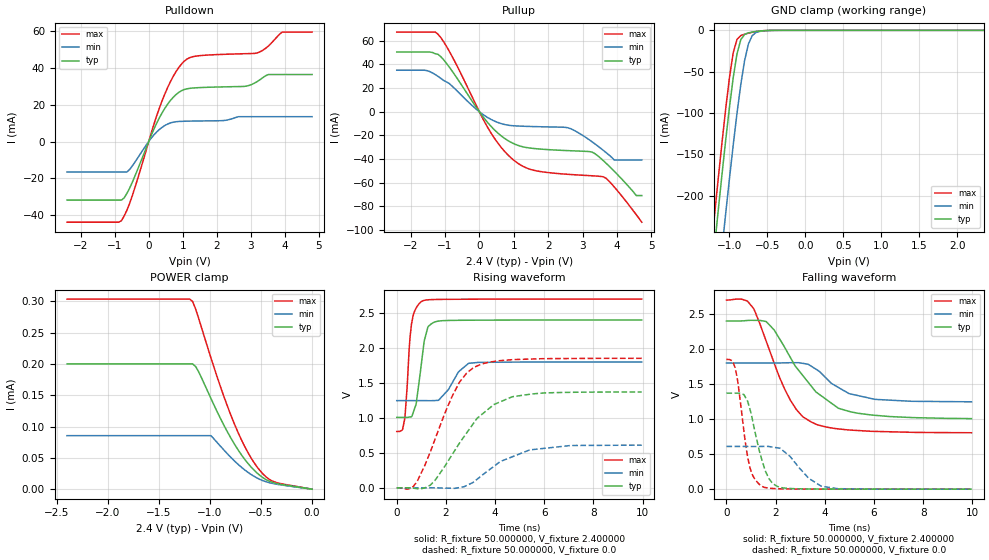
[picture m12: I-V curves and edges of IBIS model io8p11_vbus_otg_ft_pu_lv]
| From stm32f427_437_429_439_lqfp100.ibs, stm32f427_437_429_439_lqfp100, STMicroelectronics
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|   Model io8p11_vbus_otg_ft_pu_lv
[Model]  io8p11_vbus_otg_ft_pu_lv
Model_type I/O
Polarity   Non-Inverting
Enable   Active-Low
Vinl =   0.720000V
Vinh =   1.680000V
Vmeas =  1.200000V
Cref =   30.000000pF
Rref =   100.000000M
Vref =   0.0V
C_comp   3.193600pF   3.100000pF   3.332100pF
[Temperature Range]   25.000000   0.125000k   -40.000000
[Pullup Reference]   2.400000V   1.800000V   2.700000V
[Pulldown Reference]   0.0V   0.0V   0.0V
[POWER Clamp Reference]   2.400000V   1.800000V   2.700000V
[GND Clamp Reference]   0.0V   0.0V   0.0V
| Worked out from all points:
|   slope of the pulldown table from 0 to 0.36 V, typ, clamps not added: 25 ohm
|   slope of the pullup table from 0 to 0.36 V, typ, clamps not added: 27.7 ohm
|   GND clamp passes 1 mA (typ) near -0.61 V on its own axis
|   rising waveform, R_fixture 50.000000, V_fixture 2.400000: 20-80 % time 311ps typ, 636ps min, 224ps max; typ from 1.01 V to 2.4 V
|   rising waveform, R_fixture 50.000000, V_fixture 0.0: 20-80 % time 1.73ns typ, 1.75ns min, 1.31ns max; typ from 0.001 V to 1.37 V
|   falling waveform, R_fixture 50.000000, V_fixture 2.400000: 20-80 % time 1.84ns typ, 1.32ns min, 1.36ns max; typ from 2.4 V to 1.01 V
|   falling waveform, R_fixture 50.000000, V_fixture 0.0: 20-80 % time 577ps typ, 977ps min, 436ps max; typ from 1.37 V to 0.001 V
[Pulldown]
|Voltage   I(typ)   I(min)   I(max)
-2.4V     -31.69mA   -16.5mA    -43.66mA
-800mV    -31.69mA   -16.5mA    -42.82mA
-480mV    -21.96mA   -13.17mA   -29.19mA
80mV      3.63mA     1.966mA    5.014mA
480mV     18.16mA    8.738mA    26.02mA
800mV     25.38mA    10.72mA    37.77mA
1.12V     28.53mA    11.02mA    44.6mA
2.8V      29.84mA    13.46mA    47.53mA
3.2V      32.6mA     13.46mA    48.03mA
3.52V     36.28mA    13.46mA    51.75mA
3.92V     36.28mA    13.46mA    59.24mA
4.8V      36.28mA    13.46mA    59.24mA
[Pullup]
|Voltage   I(typ)   I(min)   I(max)
-2.4V     50.44mA    35.08mA    67.32mA
-1.52V    50.44mA    34.74mA    67.32mA
-1.2V     48.5mA     29.88mA    65.48mA
320mV     -11.75mA   -6.207mA   -17.08mA
1.04V     -27.53mA   -11.97mA   -41.91mA
1.6V      -31.13mA   -12.57mA   -49.63mA
2.56V     -32.88mA   -13.49mA   -52.9mA
3.28V     -34.19mA   -25.52mA   -54.18mA
3.6V      -41.31mA   -32.62mA   -54.98mA
3.92V     -50.32mA   -40.8mA    -63.62mA
4.56V     -70.9mA    -40.8mA    -87.07mA
4.72V     -70.9mA    -40.8mA    -93.4mA
[GND_clamp]
|Voltage   I(typ)   I(min)   I(max)
-2.4V     -1.424A    -1.508A    -1.393A
-1.25V    -311.3mA   -401.9mA   -273.4mA
-1.2V     -265.5mA   -356.1mA   -227.3mA
-1.15V    -220.5mA   -310.9mA   -182mA
-1.1V     -176.4mA   -266.2mA   -138mA
-1.05V    -133.9mA   -222.5mA   -96.06mA
-950mV    -57.51mA   -139mA     -27.35mA
-900mV    -28.55mA   -100.5mA   -11.03mA
-850mV    -11.33mA   -65.67mA   -6.322mA
-750mV    -3.069mA   -16.69mA   -3.425mA
-600mV    -864.6uA   -1.294mA   -852.2uA
2.35V     0A         0A         0A
[POWER_clamp]
|Voltage   I(typ)   I(min)   I(max)
-2.4V     200uA      85.42uA    303.5uA
-1.2V     200uA      85.42uA    303.5uA
-1.17V    200uA      85.42uA    299.5uA
-1.14V    195.7uA    85.42uA    287.5uA
-990mV    144.6uA    85.42uA    209.3uA
-870mV    104.1uA    63.64uA    150.8uA
-780mV    77.28uA    48.22uA    111.8uA
-660mV    47.71uA    30.77uA    68.21uA
-570mV    30.64uA    20.64uA    42.8uA
-480mV    18.19uA    13.46uA    24.07uA
-390mV    10.91uA    9.255uA    13.01uA
0V        0A         0A         0A
[Ramp]
| variable   typ   min   max
dV/dt_r  0.82171/1.73008n   0.36497/1.74767n   1.11077/1.30881n
dV/dt_f  0.83202/1.83382n   0.33210/1.34052n   1.13534/1.35770n
R_load = 50.000000
[Rising Waveform]
R_fixture= 50.000000
V_fixture= 2.400000
V_fixture_min= 1.800000
V_fixture_max= 2.700000
|time   V(typ)   V(min)   V(max)
0s        1.007V     1.247V     805.7mV
320.3ps   1.007V     1.247V     978.4mV
540.5ps   1.014V     1.247V     2.149V
620.6ps   1.026V     1.247V     2.378V
800.8ps   1.227V     1.247V     2.578V
1.021ns   1.826V     1.247V     2.667V
1.261ns   2.291V     1.247V     2.689V
1.682ns   2.384V     1.251V     2.694V
2.923ns   2.397V     1.78V      2.697V
9.97ns    2.4V       1.8V       2.699V
[Rising Waveform]
R_fixture= 50.000000
V_fixture= 0.0
V_fixture_min= 0.0
V_fixture_max= 0.0
|time   V(typ)   V(min)   V(max)
0s        1.051mV    906.3uV    1.406mV
560.6ps   -1.07mV    889uV      -7.044mV
840.8ps   -11.79mV   892.7uV    98.35mV
1.361ns   38.07mV    925.9uV    509.7mV
2.282ns   490.2mV    -6.145mV   1.329V
2.563ns   645.6mV    5.341mV    1.515V
3.123ns   922.5mV    81.83mV    1.718V
3.964ns   1.193V     310.8mV    1.808V
5.405ns   1.338V     542.2mV    1.841V
9.97ns    1.371V     610.1mV    1.852V
[Falling Waveform]
R_fixture= 50.000000
V_fixture= 2.400000
V_fixture_min= 1.800000
V_fixture_max= 2.700000
|time   V(typ)   V(min)   V(max)
0s        2.4V       1.8V       2.699V
680.7ps   2.402V     1.8V       2.705V
1.101ns   2.41V      1.8V       2.58V
1.622ns   2.391V     1.8V       2.108V
2.382ns   2.015V     1.803V     1.419V
2.843ns   1.738V     1.805V     1.138V
3.443ns   1.474V     1.757V     960.6mV
4.545ns   1.158V     1.454V     860.8mV
5.005ns   1.109V     1.363V     844.8mV
9.97ns    1.007V     1.247V     805.7mV
[Falling Waveform]
R_fixture= 50.000000
V_fixture= 0.0
V_fixture_min= 0.0
V_fixture_max= 0.0
|time   V(typ)   V(min)   V(max)
0s        1.371V     610.1mV    1.852V
240.2ps   1.371V     610.2mV    1.832V
360.4ps   1.371V     610.2mV    1.724V
860.9ps   1.257V     610mV      461.2mV
1.041ns   1.021V     609.8mV    217mV
1.441ns   420.4mV    610.1mV    41.87mV
1.722ns   155.7mV    610mV      14.87mV
2.042ns   46.2mV     592.2mV    8.041mV
3.864ns   3.013mV    43.41mV    2.226mV
9.97ns    1.051mV    906.3uV    1.406mV
